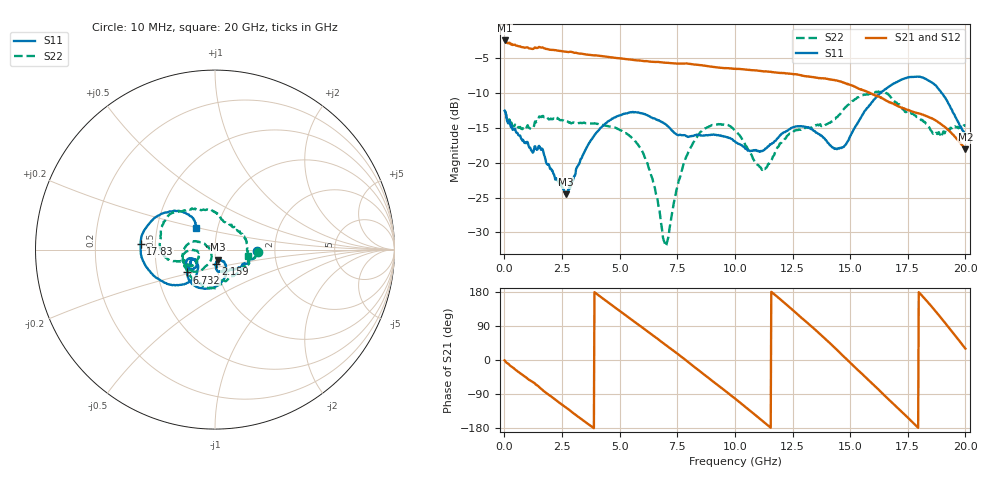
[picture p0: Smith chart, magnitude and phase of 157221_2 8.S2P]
!  2-Port S-parameters saved by WinCal
! VAR MeasName=S-Parameters (CALIBRATED_DATA) read from VNA (N5242A)
! VAR MeasDate=2015-5-26 16:47:42
! VAR NAME=157221_2 8
! VAR FILENAME=157221_2 8.S2P
! VAR DATE=2015-5-26 16:47:43
! VAR PHYS_PORTS=1,2
# Hz S DB R 50
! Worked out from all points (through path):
!   801 points, 10 MHz to 20 GHz, reference 50 ohm
!   highest |S21| = -2.41 dB at 10 MHz (marker M1); lowest = -18.1 dB at 20 GHz (marker M2)
!   group delay of S21, straight-line fit = 141 ps
!   lowest |S11| = -24.5 dB at 2.659 GHz (marker M3), VSWR 1.13, Z = 51.4 - j5.87 ohm
!   |S11| at or under -10 dB: start of sweep to 16.3 GHz; 18.98 GHz to end of sweep
!   |S22| runs from -32.0 to -9.7 dB; largest |S21 - S12| = 0.0077
!   S11 on the Smith chart (normalised r, x): 10 MHz: 1.62, -0.03; 2.159 GHz: 0.99, -0.16; 6.732 GHz: 0.71, -0.19; 17.83 GHz: 0.41, +0.03; 20 GHz: 0.79, +0.20
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1e7  -12.51 -2.1  -2.41 -0.9  -2.41 -0.8  -12.43 -2.7
1.059475e9  -17.63 -60.2  -3.53 -51.8  -3.53 -51.9  -14.96 -74.3
2.158925e9  -21.72 -87.8  -3.78 -102.3  -3.78 -102.4  -13.69 -120.5
2.658675e9  -24.53 -73.4  -4.03 -124.9  -4.03 -125.0  -14.01 -135.0
3.358325e9  -19.29 -56.2  -4.32 -156.7  -4.31 -156.9  -14.28 -150.0
4.2079e9  -14.90 -76.5  -4.64 165.2  -4.64 165.1  -14.54 -163.0
5.182412e9  -12.95 -104.1  -5.04 121.4  -5.02 121.1  -15.59 174.9
5.982012e9  -12.89 -127.9  -5.34 85.6  -5.34 85.4  -18.34 157.0
6.681662e9  -13.88 -139.7  -5.50 54.2  -5.47 54.0  -26.15 157.0
6.731638e9  -13.96 -140.5  -5.53 51.9  -5.49 51.7  -26.90 159.0
7.031488e9  -14.55 -146.1  -5.61 38.3  -5.60 38.0  -31.80 -156.6
8.155925e9  -16.14 -146.4  -5.84 -14.2  -5.84 -14.6  -17.33 -123.5
1.0005e10  -16.91 -155.9  -6.48 -101.8  -6.48 -102.3  -15.35 -173.4
1.110445e10  -18.34 -146.1  -6.80 -156.1  -6.75 -156.6  -20.64 -170.1
1.165418e10  -17.14 -136.9  -6.96 176.2  -6.93 175.7  -19.06 -150.4
1.335332e10  -15.20 -157.7  -7.67 86.9  -7.63 86.7  -14.87 -160.6
1.482759e10  -17.30 -133.1  -8.60 3.2  -8.56 2.8  -11.94 -165.8
1.58021e10  -11.87 -131.3  -9.89 -53.2  -9.79 -54.1  -10.14 166.9
1.667666e10  -9.05 -151.8  -11.24 -104.4  -11.19 -104.7  -10.25 137.7
1.782609e10  -7.64 175.6  -12.78 -171.4  -12.72 -172.9  -13.19 94.2
1.892554e10  -9.74 139.1  -14.39 112.3  -14.38 111.7  -15.72 50.0
2e10  -15.87 131.1  -18.05 30.0  -18.11 28.9  -14.65 -11.2
